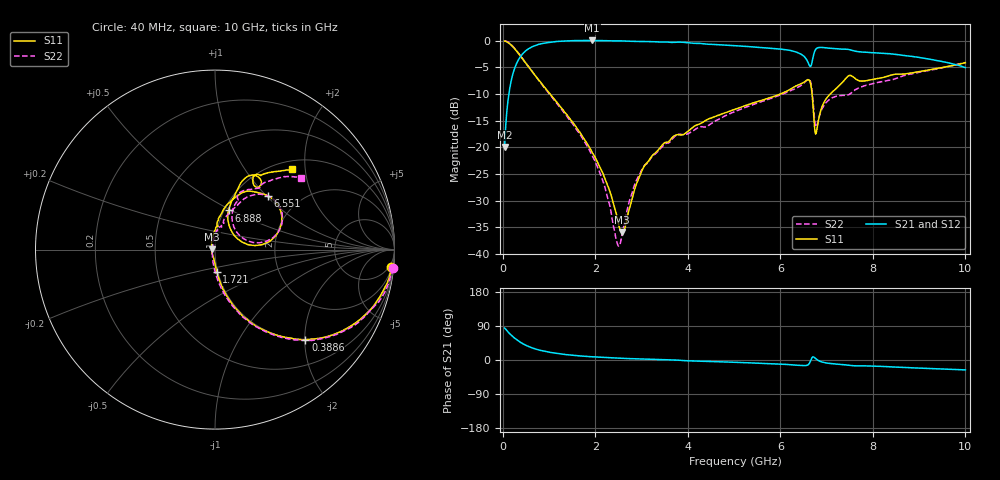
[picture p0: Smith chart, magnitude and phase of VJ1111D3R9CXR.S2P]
! VJ1111D3R9CXR
! DATE 03/04/2022  14:15
! CAPACITORS MOUNTED IN SERIES ON 25 MIL THICK MICROSTRIP SUBSTRATE
# GHz  S  MA  R  50.00
!  FREQ  S11M  S11A  S21M  S21A  S12M  S12A  S22M  S22A
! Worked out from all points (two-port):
!   801 points, 40 MHz to 10 GHz, reference 50 ohm
!   highest |S21| = 0.01 dB at 1.932 GHz (marker M1); lowest = -19.9 dB at 40 MHz (marker M2)
!   |S21| within 3 dB of the highest: 383.9 MHz to 6.516 GHz (6.132 GHz wide, 178 % of centre); 6.711 GHz to 8.856 GHz (2.145 GHz wide, 27.6 % of centre)
!   lowest |S11| = -35.9 dB at 2.58 GHz (marker M3), VSWR 1.03, Z = 48.4 + j0.2 ohm
!   |S11| at or under -10 dB: 1.021 GHz to 6.007 GHz (4.985 GHz wide, 142 % of centre); 6.685 GHz to 7.082 GHz (397.2 MHz wide, 5.77 % of centre)
!   |S22| runs from -38.5 to 0.0 dB; largest |S21 - S12| = 0.0069
!   S11 on the Smith chart (normalised r, x): 40 MHz: 2, -20; 388.6 MHz: 0.99, -2.02; 1.721 GHz: 0.99, -0.25; 6.551 GHz: 1.40, +1.02; 6.888 GHz: 1.05, +0.48; 10 GHz: 1.17, +1.70
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0.04  0.9878 -5.6  0.1007 84.3  0.1007 83.5  0.9973 -6.0
0.17695  0.9101 -23.8  0.4092 66.5  0.4091 66.8  0.9157 -23.8
0.3886  0.7111 -44.9  0.7136 46.2  0.7166 46.0  0.7149 -45.1
0.84925  0.3893 -68.0  0.937 24.4  0.9403 24.3  0.3851 -68.9
1.7083  0.1299 -84.9  1 10.4  1.006 10.3  0.1239 -89.5
1.72075  0.1272 -85.2  1 10.3  1.005 10.2  0.1221 -89.9
1.9324  0.08963 -89.2  1.001 8.5  1.005 8.3  0.08355 -95.7
2.2063  0.05115 -97.3  0.9968 6.5  1.002 6.3  0.04248 -109.6
2.46775  0.02251 -138.9  0.9913 5.2  0.9957 5.0  0.01288 -173.3
2.5798  0.01607 172.6  0.9916 4.5  0.9963 4.4  0.01547 137.4
2.8786  0.04408 116.8  0.9806 3.2  0.9854 3.0  0.04776 101.9
3.36415  0.09486 93.8  0.969 1.1  0.9736 1.0  0.09262 87.2
5.02  0.2267 77.9  0.8947 -6.1  0.8988 -6.2  0.216 69.0
6.12805  0.3334 66.5  0.8189 -11.6  0.822 -11.8  0.3255 60.2
6.55135  0.4193 45.7  0.6792 -14.6  0.6819 -14.8  0.4158 46.7
6.62605  0.4242 30.1  0.5871 -9.0  0.5892 -9.1  0.4318 32.3
6.6883  0.3072 8.5  0.6351 6.9  0.638 6.7  0.3289 11.5
6.77545  0.1364 46.5  0.8372 2.5  0.8409 2.3  0.1553 39.1
6.8875  0.2307 70.9  0.8621 -4.7  0.8655 -4.9  0.2228 64.5
7.47265  0.4666 62.9  0.8246 -14.0  0.8285 -14.2  0.3104 66.0
8.34415  0.4673 62.0  0.7526 -17.8  0.7568 -17.9  0.4237 54.4
10  0.6195 46.1  0.5569 -26.1  0.5596 -26.4  0.6216 39.8
